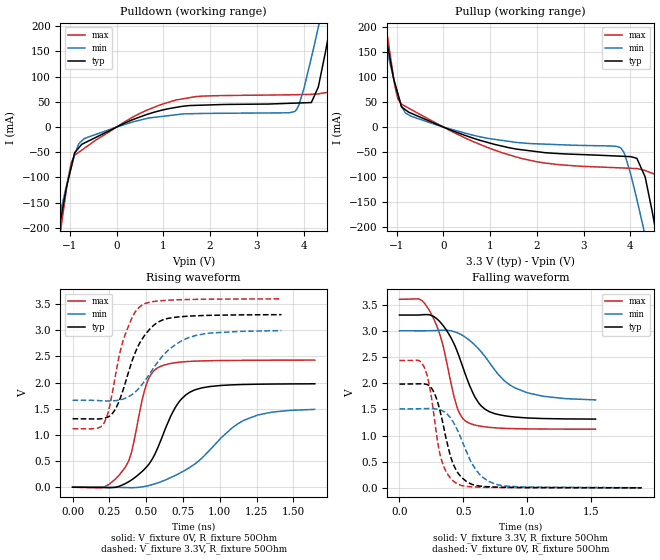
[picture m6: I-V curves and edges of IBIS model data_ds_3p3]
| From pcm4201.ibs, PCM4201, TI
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|   data_ds_3p3 Model
[Model]   data_ds_3p3
Model_type   Output
Polarity   Non-Inverting
Vmeas = 1.65
Vref = 1.65
Cref = 2pF
Rref = 50
|   typ   min   max
|   (nom PVT)   (fast PVT)   (slow PVT)
|C_comp from frequency sweep method (F=13.83MHz)
|C_comp   1.247e-12   1.127e-12   1.444e-12
|ON state : BUFFER OUTPUT TURNED HIGH
|C_comp   1.247e-12   1.127e-12   1.444e-12
|OFF state: BUFFER OUTPUT TURNED LOW
|C_comp   1.271e-12   1.187e-12   1.443e-12
|C_comp from LC tank measurement(L=1nH)
|Resonant Frequency(Hz)   7.720e+09   7.770e+09   7.490e+09
C_comp   4.254e-13   4.200e-13   4.520e-13
|ON state : BUFFER OUTPUT TURNED HIGH
|Resonant Frequency(Hz)   7.720e+09   7.770e+09   7.490e+09
|C_comp   4.254e-13   4.200e-13   4.520e-13
|OFF state: BUFFER OUTPUT TURNED LOW
|Resonant Frequency(Hz)   7.740e+09   7.900e+09   7.470e+09
|C_comp   4.232e-13   4.063e-13   4.544e-13
| Where nom  PVT is Nominal Process, 3.3V, 35C
|   Fast PVT is Strong Process,  3.6V, -10C
|   Slow PVT is Weak Process,   3V, 80C
[Voltage Range]   3.3   3   3.6
|Ambient Temperature   25   70   -10
|Junction Temperature
[Temperature Range]   35   80   -10
[Pullup Reference]   3.3   3   3.6
[Pulldown Reference]   0   0   0
[Power Clamp Reference]   3.3   3   3.6
[GND Clamp Reference]   0   0   0
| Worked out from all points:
|   slope of the pulldown table from 0 to 0.495 V, typ, clamps not added: 25 ohm
|   slope of the pullup table from 0 to 0.495 V, typ, clamps not added: 28.1 ohm
|   falling waveform, V_fixture 3.3V, R_fixture 50Ohm: 20-80 % time 203ps typ, 294ps min, 152ps max; typ from 3.3 V to 1.31 V
|   rising waveform, V_fixture 0V, R_fixture 50Ohm: 20-80 % time 206ps typ, 365ps min, 121ps max; typ from 0 V to 1.98 V
|   rising waveform, V_fixture 3.3V, R_fixture 50Ohm: 20-80 % time 164ps typ, 238ps min, 127ps max; typ from 1.31 V to 3.3 V
|   falling waveform, V_fixture 0V, R_fixture 50Ohm: 20-80 % time 127ps typ, 180ps min, 101ps max; typ from 1.98 V to 0.002 V
[Pulldown]
|   Voltage   I(typ)   I(min)   I(max)
-3.3V     -1.347A    -1.084A    -1.741A
-1.328V   -252.6mA   -221.6mA   -291.5mA
-1.104V   -136.2mA   -129.5mA   -144.6mA
-968.4mV  -79.09mA   -79.59mA   -70.65mA
-804mV    -40.75mA   -32.57mA   -49.7mA
18mV      811.1uA    603.1uA    1.128mA
1.289V    39.28mA    24.6mA     53.95mA
3.81V     47.47mA    30.76mA    64.08mA
4.316V    79.27mA    198.1mA    65.81mA
4.586V    209.9mA    313.8mA    74.95mA
4.867V    359.1mA    437.4mA    226.8mA
6.6V      1.329A     1.2A       1.496A
[Pullup]
|   Voltage   I(typ)   I(min)   I(max)
-3.3V     1.329A     1.068A     1.72A
-1.314V   224.1mA    197.1mA    257.3mA
-975.6mV  66.67mA    67.2mA     56.95mA
-693mV    27.81mA    21.83mA    35.24mA
1.559V    -44.06mA   -30.77mA   -59.99mA
3.786V    -58.33mA   -41.27mA   -81.72mA
4.138V    -62.58mA   -144.5mA   -83.06mA
4.314V    -99.37mA   -216.3mA   -86.96mA
4.511V    -191.4mA   -299.6mA   -94.31mA
4.59V     -233.5mA   -333.5mA   -102.1mA
4.871V    -382.5mA   -456.2mA   -254.8mA
6.6V      -1.347A    -1.218A    -1.518A
[Ramp]
R_load = 50
|   typ   min   max
dV/dt_r   1.18677/2.05737e-10   0.898443/3.66884e-10   1.45787/1.20573e-10
dV/dt_f   1.19339/2.02217e-10   0.799076/2.97701e-10   1.48821/1.51631e-10
[Falling Waveform]
V_fixture = 3.3V
V_fixture_min = 3V
V_fixture_max = 3.6V
R_fixture = 50Ohm
|   Time   V(typ)   V(min)   V(max)
0s        3.3V       3V         3.6V
159ps     3.302V     2.999V     3.601V
237.5ps   3.303V     3.001V     3.375V
334ps     3.125V     3.01V      2.79V
451ps     2.62V      2.965V     1.549V
530.5ps   2.079V     2.853V     1.256V
593ps     1.731V     2.723V     1.199V
672.5ps   1.501V     2.503V     1.165V
907ps     1.352V     1.908V     1.131V
1.538ns   1.313V     1.68V      1.121V
[Rising Waveform]
V_fixture = 0V
V_fixture_min = 0V
V_fixture_max = 0V
R_fixture = 50Ohm
|   Time   V(typ)   V(min)   V(max)
0s        738.5pV    1.224nV    535pV
214ps     -5.993mV   571.6uV    3.665mV
356ps     65.55mV    -5.948mV   373.1mV
402ps     141.8mV    -8.747mV   686.4mV
503ps     387.5mV    22.25mV    1.976V
592ps     844mV      95.95mV    2.302V
713ps     1.589V     247mV      2.384V
832ps     1.86V      446.8mV    2.409V
1.165ns   1.963V     1.28V      2.424V
1.645ns   1.976V     1.487V     2.429V
[Rising Waveform]
V_fixture = 3.3V
V_fixture_min = 3V
V_fixture_max = 3.6V
R_fixture = 50Ohm
|   Time   V(typ)   V(min)   V(max)
0s        1.308V     1.661V     1.118V
216.5ps   1.318V     1.65V      1.237V
251ps     1.358V     1.648V     1.535V
291ps     1.489V     1.654V     2.131V
344ps     1.864V     1.685V     2.806V
404ps     2.411V     1.771V     3.236V
461.5ps   2.781V     1.924V     3.458V
585ps     3.16V      2.414V     3.559V
788.5ps   3.268V     2.856V     3.586V
1.419ns   3.296V     2.992V     3.598V
[Falling Waveform]
V_fixture = 0V
V_fixture_min = 0V
V_fixture_max = 0V
R_fixture = 50Ohm
|   Time   V(typ)   V(min)   V(max)
0s        1.982V     1.508V     2.431V
192ps     1.986V     1.514V     2.317V
241.5ps   1.933V     1.515V     1.867V
296.5ps   1.661V     1.501V     928.4mV
327.5ps   1.376V     1.48V      552.1mV
400ps     607.6mV    1.339V     187.3mV
456ps     295.2mV    1.096V     74.67mV
598ps     47.73mV    351.2mV    16.58mV
752.5ps   15.85mV    71.85mV    7.567mV
1.899ns   1.663mV    2.613mV    1.026mV
